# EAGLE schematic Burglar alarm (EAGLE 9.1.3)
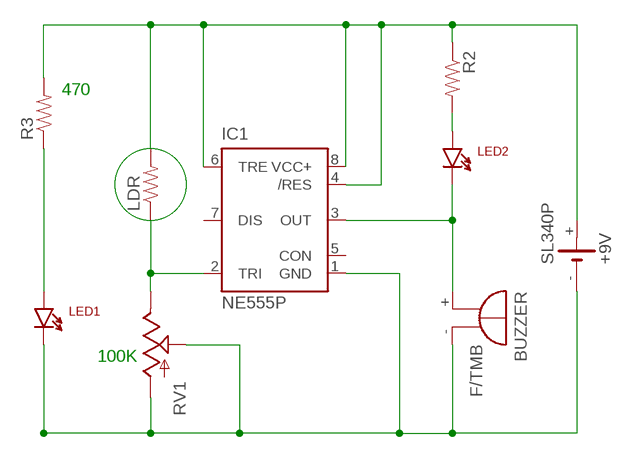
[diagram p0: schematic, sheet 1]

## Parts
+9V  SL340P  [SL-340/P3.6V]
BUZZER  F/TMB  [F/TMB]
IC1  NE555P  [DIL-08]
LDR  RESISTORAXIAL-0.3  [AXIAL-0.3]
LED1  LTE-302  [LTE-302]
LED2  LTE-302  [LTE-302]
R2  RESISTORAXIAL-0.3  [AXIAL-0.3]
R3  RESISTORAXIAL-0.3  [AXIAL-0.3]
RV1  POTTRIM  [TRIM_POT]

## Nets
N$1: IC1.2(TRI) LDR.P$1 RV1.2(E)
N$2: BUZZER.+ IC1.3(OUT) LED2.C
N$3: LED2.A R2.P$2
N$4: LED1.A R3.P$1
N$5: +9V.+ IC1.4(/RES) IC1.6(TRE) IC1.8(VCC+) LDR.P$2 R2.P$1 R3.P$2
N$6: +9V.- BUZZER.- IC1.1(GND) LED1.C RV1.1(S) RV1.3(A)
Unconnected: IC1.5(CON) IC1.7(DIS)

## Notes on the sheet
- 470
- 100K

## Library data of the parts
+9V = battery:SL340P: LI BATTERY Sonnenschein
BUZZER = buzzer:F/TMB: BUZZER; OC_FARNELL: unknown; OC_NEWARK: unknown
IC1 = SparkFun-AnalogIC:NE555: General purpose bipolar Timer; MF: Arrow Electronics; MPN: NE555N; OC_FARNELL: 1467742; OC_NEWARK: 89K1486
LDR R2 R3 = SparkFun-Passives:RESISTOR: Resistor
LED1 LED2 = SparkFun-LED:LTE-302: Through-hole side-firing 940nm IR LED
RV1 = SparkFun-Retired:POT; PROD_ID: COM-00104

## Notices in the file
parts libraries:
SparkFun-AnalogIC: Licensing: CC v3.0 Share-Alike You are welcome to use this library for commercial purposes.
SparkFun-Retired: Licensing: Creative Commons ShareAlike 4.0 International - https://creativecommons.org/licenses/by-sa/4.0
